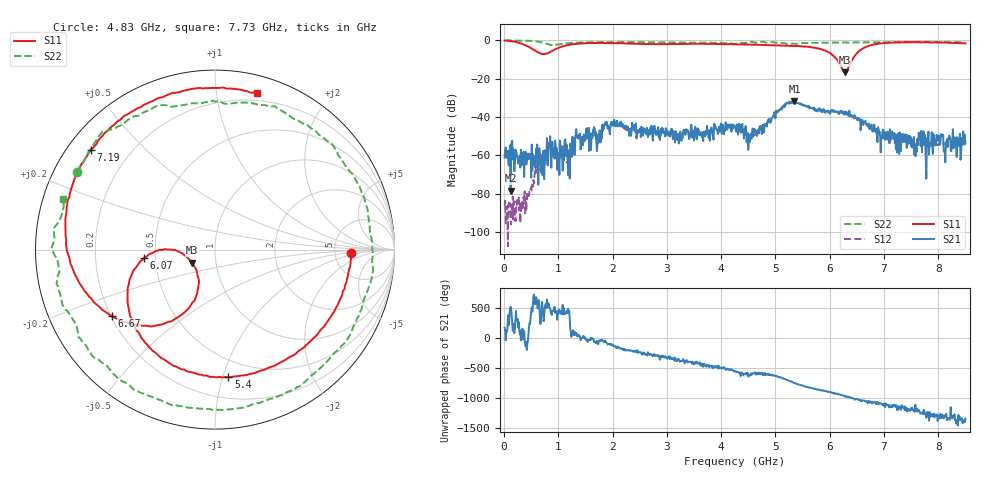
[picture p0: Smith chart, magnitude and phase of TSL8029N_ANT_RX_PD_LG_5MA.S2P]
!Agilent Technologies,E5071C,MY46523237,B.13.01
!Date: Wed Oct 18 11:30:20 2023
!Data & Calibration Information:
!Freq	S11:SOLT2(ON)	S21:SOLT2(ON)	S12:SOLT2(ON)	S22:SOLT2(ON)
!PortZ  Port1:50+j0  Port2:50+j0
!Above PortZ is port z conversion or system Z0 setting when saving the data.
!When reading, reference impedance value at option line is always used.
# Hz S dB R 50
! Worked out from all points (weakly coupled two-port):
!   850 points, 10 MHz to 8.5 GHz, reference 50 ohm
!   highest |S21| = -31.78 dB at 5.35 GHz (marker M1); lowest = -78.5 dB at 120 MHz (marker M2)
!   lowest |S11| = -16.6 dB at 6.28 GHz (marker M3), VSWR 1.35, Z = 38.2 - j5.76 ohm
!   |S11| at or under -10 dB: 6.134 GHz to 6.417 GHz (282.7 MHz wide, 4.51 % of centre)
!   |S22| runs from -2.4 to 0.0 dB; largest |S21 - S12| = 0.0039
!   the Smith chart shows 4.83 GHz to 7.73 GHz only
!   S11 on the Smith chart (normalised r, x): 4.83 GHz: 7.25, -0.74; 5.4 GHz: 0.36, -1.04; 6.07 GHz: 0.43, -0.05; 6.67 GHz: 0.20, -0.28; 7.19 GHz: 0.07, +0.35; 7.73 GHz: 0.14, +1.29
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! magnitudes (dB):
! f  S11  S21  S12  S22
! 10 MHz  0.0  -61.2  -86.5  0.0
! 120 MHz  -0.2  -78.5  -92.3  0.0
! 470 MHz  -3.6  -60.8  -78.0  -0.2
! 700 MHz  -7.0  -60.7  -65.3  -1.1
! 850 MHz  -6.0  -50.0  -54.0  -2.3
! 1.15 GHz  -2.5  -58.8  -63.6  -1.5
! 1.43 GHz  -1.5  -50.4  -52.1  -1.0
! 2 GHz  -1.4  -42.7  -43.1  -0.9
! 2.84 GHz  -1.9  -45.2  -48.2  -1.0
! 4.26 GHz  -2.0  -44.9  -44.0  -1.8
! 4.51 GHz  -2.1  -50.3  -49.9  -0.9
! 4.83 GHz  -2.4  -43.5  -43.6  -1.1
! 5.35 GHz  -2.9  -31.8  -32.1  -1.6
! 5.4 GHz  -2.9  -32.5  -32.5  -1.7
! 5.67 GHz  -3.6  -35.3  -35.3  -1.2
! 6.07 GHz  -8.0  -37.1  -37.2  -1.0
! 6.28 GHz  -16.6  -37.8  -38.1  -1.0
! 6.67 GHz  -3.3  -43.5  -44.2  -1.0
! 7.09 GHz  -1.2  -47.8  -50.7  -1.0
! 7.19 GHz  -1.1  -48.3  -51.5  -0.9
! 7.73 GHz  -0.9  -47.5  -54.3  -1.0
! 8.5 GHz  -1.5  -53.9  -54.4  -1.0
